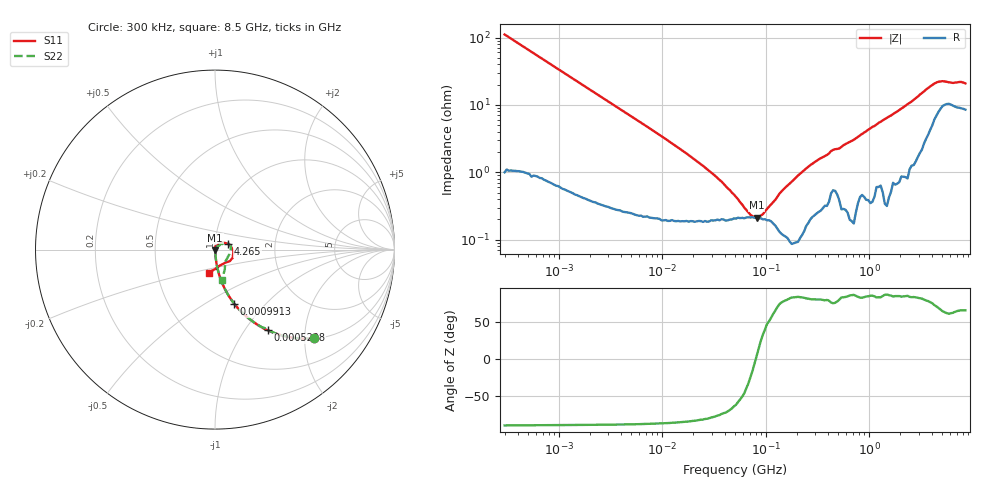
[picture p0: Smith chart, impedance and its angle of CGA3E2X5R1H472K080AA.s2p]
! S-parameter Generated by TDK Corporation
! Copyright(C) 2015 TDK Corporation.
! All Rights Reserved.
! TDK P/N: CGA3E2X5R1H472K080AA (Multilayer Ceramic Chip Capacitors)
! Property: C=4.7nF
! Size(LxWxT): 1.6x0.8x0.8mm, 0.063x0.031x0.031inches
! Model Type: s2p (Touchstone File Format Version 1.0)
! Frequency: DC=Yes Start=0.3MHz Stop=8500MHz 225points Log-sweep
! Note:
! Model Generated on Jun. 23, 2015
! Hash(MD5):
! Port Assignments:
!  1 ---| |--- 2
! Applicable Conditions:
!  Temperature = 25 degC
!  DC Bias Voltage = 0 V
!  Small Signal Operation
! Terms and conditions regarding TDK Simulation Models
! (1)This simulation model is being provided solely for informational purposes. Please refer to the specifications of the products in terms of detailed characteristics of such products.
! (2)In no event shall TDK Corporation of any of its subsidiaries be liable for any loss or damage arising, directly or indirectly,
!  From any information contained in this simulation model, including, but not limited to loss or damages arising from any inaccuracies, omissions or errors in connection with such information.
! (3)Any and all copyrights on this simulation model are owned by TDK Corporation.
!  Duplication or redistribution of this simulation model without prior written permission from TDK Corporation is prohibited.
! (4)This simulation model is subject to any modification or change without any prior notice.
! (5)Neither TDK Corporation nor any of its subsidiaries shall make any warranty, express or implied,
!  Including but not limited to the correctness, implied warranties of merchantability and fitness for a particular purpose with respect to this simulation models.
! (6)The use of this simulation model shall be deemed to have consented to the terms and conditions hereof.
# MHz S MA R 50
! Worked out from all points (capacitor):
!   224 points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, 300 kHz to 8.5 GHz, reference 50 ohm
!   read as one part in series: C = 4.77 nF near 314.1 kHz
!   lowest |Z| = 212 mohm at 81.83 MHz (marker M1)
!   series resonance near 80.1 MHz, so ESL is about 830 pH
!   S11 on the Smith chart (normalised r, x): 300 kHz: 1.01, -2.22; 520.8 kHz: 1.02, -1.28; 991.3 kHz: 1.01, -0.68; 4.265 GHz: 1.15, +0.07; 8.5 GHz: 0.90, -0.24
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0.3  0.7411 -41.8  0.6677 47.7  0.6666 48.0  0.74 -41.8
0.5208429  0.5371 -56.8  0.8365 32.4  0.8346 32.6  0.5369 -56.8
0.9913414  0.3202 -70.4  0.9428 18.6  0.9408 18.8  0.3202 -70.4
1.72111  0.1925 -77.8  0.9783 11.0  0.9767 11.2  0.1924 -77.8
9.430415  0.03622 -85.0  0.998 1.9  0.9965 2.1  0.03597 -85.1
51.67171  0.005989 -71.9  0.9983 -0.0  0.9973 0.2  0.00604 -70.6
81.82903  0.002505 -47.9  0.9981 -0.3  0.9971 -0.1  0.004334 -62.5
148.7505  0.0007748 120.3  0.9985 -0.8  0.9973 -0.5  0.001228 -45.7
170.7477  0.001146 147.1  0.9981 -0.9  0.9969 -0.6  0.0002449 171.2
178.7805  0.001175 153.3  0.998 -0.9  0.9969 -0.7  0.0007784 137.8
195.9978  0.001136 158.9  0.9977 -1.0  0.9965 -0.8  0.001916 121.1
283.1228  0.002216 72.9  0.9968 -1.4  0.9956 -1.2  0.004876 80.4
373.0505  0.002483 38.8  0.9962 -1.8  0.9952 -1.6  0.007015 68.6
448.3627  0.008468 47.3  0.9949 -2.2  0.9941 -1.9  0.007229 40.9
618.5683  0.008085 92.5  0.9954 -3.0  0.9944 -2.7  0.001825 59.9
743.4462  0.002919 102.3  0.9946 -3.5  0.9935 -3.2  0.007274 92.0
853.3868  0.007903 59.4  0.9943 -3.9  0.9935 -3.7  0.007147 61.8
1124.446  0.006032 70.5  0.9933 -5.2  0.9921 -4.9  0.01087 75.9
1415.031  0.01726 86.5  0.993 -6.5  0.9919 -6.2  0.008168 82.0
1551.304  0.01164 86.9  0.992 -7.1  0.991 -6.8  0.01341 76.7
4265.177  0.078 24.2  0.9383 -19.6  0.9377 -19.2  0.08304 25.2
8500  0.1325 -104.9  0.8948 -31.9  0.8948 -31.0  0.1728 -76.6
